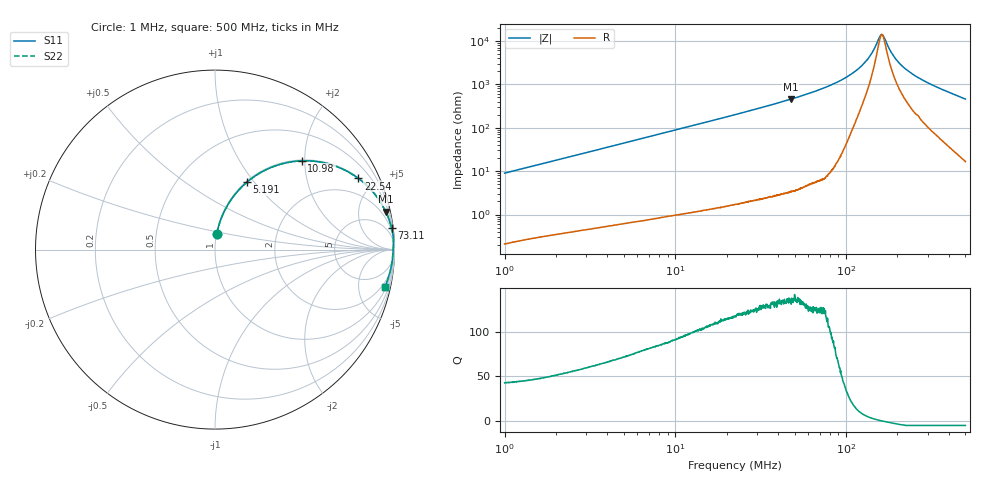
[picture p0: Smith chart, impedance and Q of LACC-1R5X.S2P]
!s-Parameter Generated by FASTRON Sdn. Bhd.
!FASTRON P/N : LACC-1R5X
!Keysight Technologies,E4991B,MY54100416,A.01.15
!Date: Wed Mar 18 08:59:52 2026
!Version  : Rev00 Wed Mar 18 08:59:52 2026
!Data & Calibration Information:
!PortZ  Port1:50+j0  Port2:50+j0
!When reading, reference impedance value at option line is always used.
!Remarks : This data is being provided solely for informational purposes.
!Freq	S11	S21	S12	S22
# Hz S dB R 50
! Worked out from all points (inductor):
!   1601 points, 1 MHz to 500 MHz, reference 50 ohm
!   read as one part in series: L = 1.42 uH near 1.032 MHz
!   highest Q = 137 at 47.32 MHz (marker M1), where L = 1.52 uH
!   self-resonance near 162.2 MHz
!   S11 on the Smith chart (normalised r, x): 1 MHz: 1.00, +0.18; 5.191 MHz: 1.01, +0.92; 10.98 MHz: 1.02, +1.94; 22.54 MHz: 1.03, +4.02; 73.11 MHz: 1, +16; 500 MHz: 1.33, -9.11
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1000000  -20.98 83.5  -0.05 -5.1  -0.05 -5.1  -20.98 83.5
2820919  -12.33 75.0  -0.30 -14.0  -0.30 -14.0  -12.33 75.0
5190713  -7.65 64.7  -0.87 -24.5  -0.87 -24.5  -7.65 64.7
7957584  -4.87 54.5  -1.79 -34.8  -1.79 -34.8  -4.87 54.5
1.098475e7  -3.20 45.6  -2.92 -43.8  -2.92 -43.8  -3.20 45.6
1.522251e7  -1.95 36.4  -4.53 -53.0  -4.53 -53.0  -1.95 36.4
2.236068e7  -1.00 26.5  -6.99 -63.0  -6.99 -63.0  -1.00 26.5
2.253506e7  -0.99 26.4  -7.05 -63.1  -7.05 -63.1  -0.99 26.4
4.732038e7  -0.22 12.5  -13.30 -77.1  -13.30 -77.1  -0.22 12.5
6.307767e7  -0.11 8.8  -16.35 -80.8  -16.35 -80.8  -0.11 8.8
7.310989e7  -0.08 7.1  -18.15 -82.4  -18.15 -82.4  -0.08 7.1
9.745486e7  -0.04 4.2  -22.69 -84.4  -22.69 -84.4  -0.04 4.2
1.211344e8  -0.04 2.3  -27.96 -81.7  -27.96 -81.7  -0.04 2.3
1.387738e8  -0.05 1.2  -33.30 -73.5  -33.30 -73.5  -0.05 1.2
1.602216e8  -0.06 0.1  -42.84 -13.6  -42.84 -13.6  -0.06 0.1
1.659216e8  -0.06 -0.2  -42.10 22.1  -42.10 22.1  -0.06 -0.2
1.77937e8  -0.07 -0.7  -36.87 57.0  -36.87 57.0  -0.07 -0.7
1.893459e8  -0.07 -1.2  -33.17 67.7  -33.17 67.7  -0.07 -1.2
2.030576e8  -0.08 -1.7  -30.14 73.1  -30.14 73.1  -0.08 -1.7
2.465825e8  -0.09 -3.3  -24.61 78.3  -24.61 78.3  -0.09 -3.3
3.299715e8  -0.13 -6.2  -19.30 79.2  -19.30 79.2  -0.13 -6.2
5e8  -0.27 -12.3  -13.45 75.6  -13.45 75.6  -0.27 -12.3
